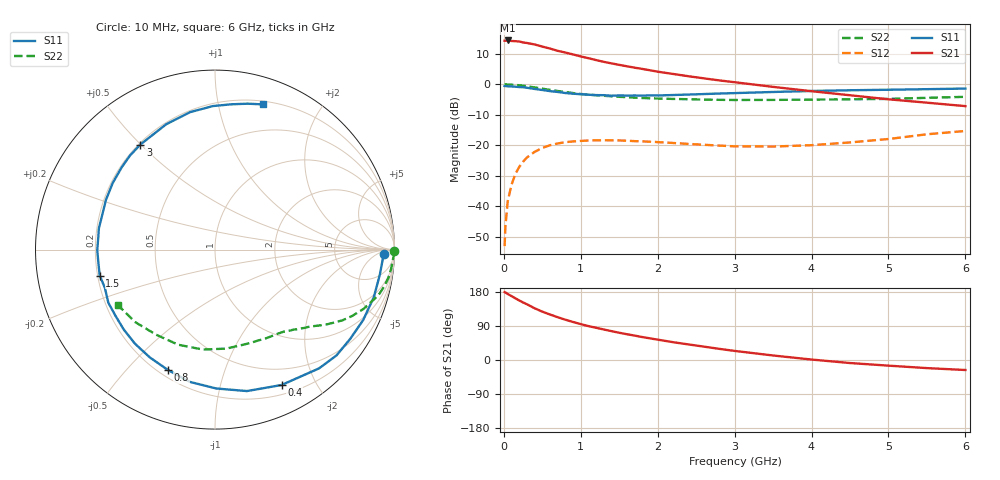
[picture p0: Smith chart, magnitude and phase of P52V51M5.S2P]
! SIEMENS Small Signal Semiconductors
! BFP183
! Si NPN RF Bipolar Junction Transistor in SOT143
! VCE = 2.5 V  IC = 1.5 mA
! Common Emitter S-Parameters:  March  1996
# GHz  S  MA  R  50
!  f  S11  S21  S12  S22
! GHz  MAG  ANG  MAG  ANG  MAG  ANG  MAG  ANG
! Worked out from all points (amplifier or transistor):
!   36 points, 10 MHz to 6 GHz, reference 50 ohm
!   highest |S21| = 14.4 dB at 50 MHz (marker M1)
!   |S21| within 3 dB of that: start of sweep to 645.5 MHz
!   unconditionally stable (mu >= 1): 2.266 GHz to 5.994 GHz
!   at 250 MHz: K = 0.11, MSG = 19.6 dB, |S12| = -25.4 dB
!   at 1.4 GHz: K = 0.61, MSG = 12.6 dB, |S12| = -18.4 dB
!   at 6 GHz: K = 1.00, MSG = 4.1 dB, |S12| = -15.3 dB
!   S11 on the Smith chart (normalised r, x): 10 MHz: 27, -12; 400 MHz: 0.30, -1.56; 800 MHz: 0.24, -0.66; 1.5 GHz: 0.21, -0.11; 3 GHz: 0.21, +0.50; 6 GHz: 0.23, +1.36
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0.01  0.9404 -1.6  5.213 179.2  0.0022 88.1  0.9998 -0.6
0.02  0.936 -3.3  5.195 178.3  0.0046 85.4  0.9995 -1.3
0.05  0.929 -8.6  5.258 174.3  0.0119 86.2  0.9929 -3.1
0.1  0.9237 -16.6  5.154 168.6  0.0225 79.5  0.9872 -6.2
0.2  0.9028 -33.4  5.059 157.1  0.044 70.9  0.9657 -12.1
0.3  0.8796 -48.8  4.776 147.1  0.0629 61.8  0.9298 -17.2
0.4  0.8407 -63.8  4.521 136.5  0.0779 54.2  0.891 -21.8
0.5  0.808 -77.3  4.172 127.6  0.0903 46.8  0.8491 -25.8
0.6  0.7738 -89.5  3.871 120.0  0.1 40.6  0.8124 -29.0
0.7  0.7503 -100.8  3.552 112.9  0.1069 35.3  0.7778 -31.5
0.8  0.7203 -111.3  3.329 106.3  0.1124 30.7  0.748 -33.9
0.9  0.7019 -121.2  3.098 100.3  0.1155 26.6  0.719 -36.0
1.1  0.6758 -138.8  2.689 89.4  0.1196 19.9  0.6763 -39.5
1.3  0.6639 -153.6  2.342 80.5  0.1208 14.3  0.6483 -42.7
1.5  0.6583 -167.3  2.089 71.9  0.1199 10.3  0.6239 -45.6
1.8  0.6537 174.8  1.792 60.5  0.1158 6.4  0.5961 -50.1
2.2  0.6679 155.4  1.481 47.0  0.1089 3.0  0.5761 -56.8
3  0.718 125.4  1.084 24.0  0.0959 5.4  0.5535 -72.5
3.5  0.7493 111.3  0.909 11.9  0.0951 11.2  0.5552 -83.6
4.5  0.8 90.8  0.662 -8.0  0.1112 22.1  0.5681 -111.1
5.5  0.8333 77.3  0.5 -21.4  0.1513 24.7  0.6009 -137.8
6  0.8522 71.7  0.439 -26.4  0.1716 21.4  0.624 -150.5
